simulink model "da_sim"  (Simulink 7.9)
settings: Solver=FixedStepDiscrete  SolverMode=SingleTasking  StartTime=0.0  StopTime=500  FixedStep=1  RelTol=1e-3  AbsTol=1e-6
PreLoadFcn:
  | init_exercise_4
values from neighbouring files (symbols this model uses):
  w = 0.1    [init_exercise_4.m]    (also in system_postloadfcn.m)
libraries: labmvlib x3

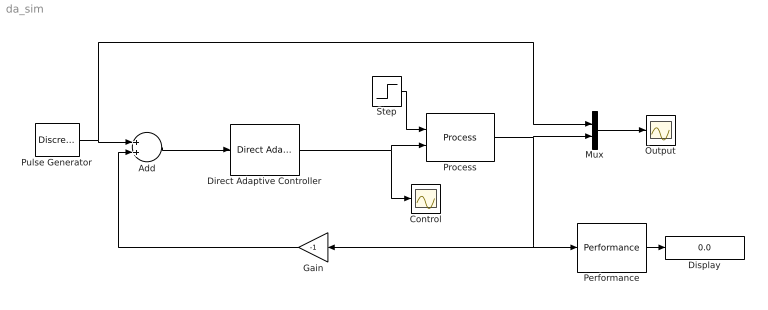
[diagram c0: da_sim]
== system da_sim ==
  Add : Sum
  Control : Scope
  Direct Adaptive Controller : labmvlib/Direct Adaptive Controller
  Display : Display
  Gain : Gain  Gain=-1  SampleTime=1
  Mux : Mux  Inputs=2
  Output : Scope
  Performance : labmvlib/Performance
  Process : labmvlib/Process
  Pulse Generator : DiscretePulseGenerator  PulseType=Time based  Amplitude=5  Period=100  PulseWidth=50
  Step : Step  Time=250  Before=w  After=10*w  SampleTime=1
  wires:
  Performance/1 -> Display/1
  Step/1 -> Process/1
  Direct Adaptive Controller/1 -> Control/1, Process/2
  Add/1 -> Direct Adaptive Controller/1
  Gain/1 -> Add/2
  Mux/1 -> Output/1
  Process/1 -> Mux/2, Performance/1, Gain/1
  Pulse Generator/1 -> Add/1, Mux/1
